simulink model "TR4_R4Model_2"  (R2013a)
settings: Solver=ode45  StartTime=0  StopTime=0.1  FixedStep=1e-4
PreLoadFcn:
  | warning('off','sm:sli:setup:compile:LocalSolverNotSupported')
InitFcn:
  |  SimParam.IC = SM2_InitCondConstrFnc(RawParam,IC);
model workspace (MAT data in the model file):
  handle : class17 (value not decoded)
  handle : class17 (value not decoded)
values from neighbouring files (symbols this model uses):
  RawParam = RobotParamGather(ParamLib)    [main_TR4.m]    (also in DeltaModelMain_v2.m; main_TimeSimulation.m; MGI.m = y)
libraries: SM2_BallJointPartsLib x8, SM2_ForeArmPartsLib x8, SM2_ArmPartsLib x4, SM2_MotorPartsLib x4, ElecDriverLib x1, SM2_FramePartsLib x1, SM2_ToolPartsLib x1

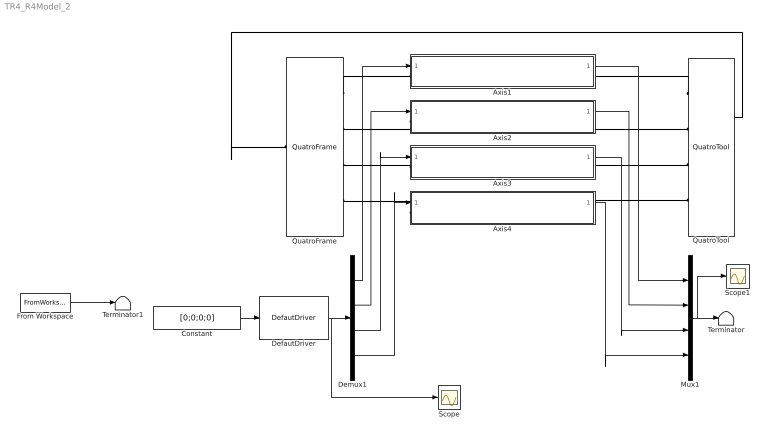
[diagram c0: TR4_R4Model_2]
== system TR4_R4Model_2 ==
  Axis1 : Subsystem
  Axis2 : Subsystem
  Axis3 : Subsystem
  Axis4 : Subsystem
  Constant : Constant  Value=[0;0;0;0]
  DefautDriver : ElecDriverLib/DefautDriver  VariantControl=driverVarDefault
  Demux1 : Demux
  From Workspace : FromWorkspace  VariableName=simin  SampleTime=0
  Mux1 : Mux
  QuatroFrame : SM2_FramePartsLib/QuatroFrame
  QuatroTool : SM2_ToolPartsLib/QuatroTool
  Scope : Scope
  Scope1 : Scope
  Terminator : Terminator
  Terminator1 : Terminator
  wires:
  Axis1/1(Alpha) -> Mux1/1
  Axis2/1(Alpha) -> Mux1/2
  Axis4/1(Alpha) -> Mux1/4
  Axis3/1(Alpha) -> Mux1/3
  Constant/1 -> DefautDriver/1
  From Workspace/1 -> Terminator1/1
  DefautDriver/1 -> Scope/1, Demux1/1
  Demux1/1 -> Axis1/1(Torque)
  Demux1/2 -> Axis2/1(Torque)
  Demux1/3 -> Axis3/1(Torque)
  Demux1/4 -> Axis4/1(Torque)
  Mux1/1 -> Scope1/1, Terminator/1
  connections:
  QuatroFrame/RConn1 -- Axis1/LConn1
  Axis2/LConn1 -- QuatroFrame/RConn2
  Axis3/LConn1 -- QuatroFrame/RConn3
  Axis3/RConn1 -- QuatroTool/RConn3
  Axis2/RConn1 -- QuatroTool/RConn2
  QuatroTool/RConn1 -- Axis1/RConn1
  QuatroTool/LConn1 -- QuatroFrame/LConn1
  Axis4/LConn1 -- QuatroFrame/RConn4
  Axis4/RConn1 -- QuatroTool/RConn4

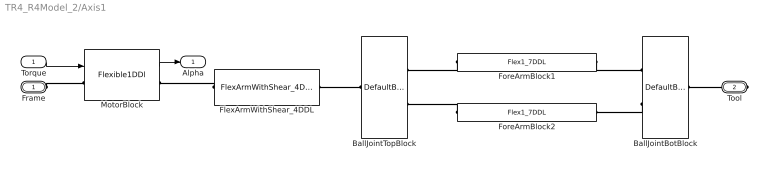
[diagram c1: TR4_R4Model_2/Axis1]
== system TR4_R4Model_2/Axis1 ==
  Torque : Inport
  BallJointBotBlock : SM2_BallJointPartsLib/DefaultBallJointBotPair
  BallJointTopBlock : SM2_BallJointPartsLib/DefaultBallJointTopPair
  FlexArmWithShear_4DDL : SM2_ArmPartsLib/FlexArmWithShear_4DDL  VariantControl=armVarFlex1_2ddl
  ForeArmBlock1 : SM2_ForeArmPartsLib/Flex1_7DDL  VariantControl=foreArmVarFlex1_7ddl
  ForeArmBlock2 : SM2_ForeArmPartsLib/Flex1_7DDL  VariantControl=foreArmVarFlex1_7ddl
  MotorBlock : SM2_MotorPartsLib/Flexible1DDl  VariantControl=motorVarFlex1
      link override Revolute Joint: ClassName=RevoluteJoint  SenseConstraintForceX=off  SenseConstraintForceY=off  SenseConstraintForceZ=off  SenseConstraintTorqueX=off  SenseConstraintTorqueY=off  SenseConstraintTorqueZ=off  ConstraintWrenchDir=FollowerOnBase  ConstraintWrenchFrame=BaseFrame  EquilibriumPosition=SimParam.Motor.Alpha(AxisID)  EquilibriumPositionUnits=rad  SpringStiffness=SimParam.Motor.kSup  SpringStiffnessUnits=N*m/rad  DampingCoefficient=SimParam.Motor.c  DampingCoefficientUnits=N*m/(rad/s)  ActuationMode=TorqueForceActuation  SensePosition=on  SenseVelocity=off  SenseAcceleration=off  SenseTorqueForce=off  PositionTargetValue=SimParam.Motor.Alpha(AxisID)  PositionTargetValueUnits=rad  PositionTargetSpecify=on  PositionTargetPriority=High  VelocityTargetValue=0  VelocityTargetValueUnits=rad/s  VelocityTargetSpecify=on  VelocityTargetPriority=High  BlockFunction=simmechanics.library.joints.revolute_joint
  Frame : PMIOPort  Port=1  Side=Left
  Tool : PMIOPort  Port=2  Side=Right
  Alpha : Outport
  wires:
  Torque/1 -> MotorBlock/1
  MotorBlock/1 -> Alpha/1
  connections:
  FlexArmWithShear_4DDL/LConn1 -- MotorBlock/RConn1
  Frame/RConn1 -- MotorBlock/LConn1
  FlexArmWithShear_4DDL/RConn1 -- BallJointTopBlock/RConn1
  Tool/RConn1 -- BallJointBotBlock/RConn1
  ForeArmBlock2/LConn1 -- BallJointTopBlock/LConn2
  ForeArmBlock1/LConn1 -- BallJointTopBlock/LConn1
  ForeArmBlock1/RConn1 -- BallJointBotBlock/LConn1
  BallJointBotBlock/LConn2 -- ForeArmBlock2/RConn1

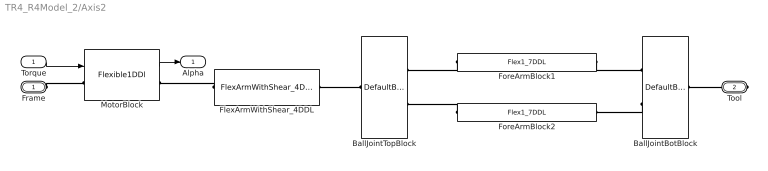
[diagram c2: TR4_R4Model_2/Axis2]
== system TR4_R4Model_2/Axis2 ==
  Torque : Inport
  BallJointBotBlock : SM2_BallJointPartsLib/DefaultBallJointBotPair
  BallJointTopBlock : SM2_BallJointPartsLib/DefaultBallJointTopPair
  FlexArmWithShear_4DDL : SM2_ArmPartsLib/FlexArmWithShear_4DDL  VariantControl=armVarFlex1_2ddl
  ForeArmBlock1 : SM2_ForeArmPartsLib/Flex1_7DDL  VariantControl=foreArmVarFlex1_7ddl
  ForeArmBlock2 : SM2_ForeArmPartsLib/Flex1_7DDL  VariantControl=foreArmVarFlex1_7ddl
  MotorBlock : SM2_MotorPartsLib/Flexible1DDl  VariantControl=motorVarFlex1
      link override Revolute Joint: ClassName=RevoluteJoint  SenseConstraintForceX=off  SenseConstraintForceY=off  SenseConstraintForceZ=off  SenseConstraintTorqueX=off  SenseConstraintTorqueY=off  SenseConstraintTorqueZ=off  ConstraintWrenchDir=FollowerOnBase  ConstraintWrenchFrame=BaseFrame  EquilibriumPosition=SimParam.Motor.Alpha(AxisID)  EquilibriumPositionUnits=rad  SpringStiffness=SimParam.Motor.kSup  SpringStiffnessUnits=N*m/rad  DampingCoefficient=SimParam.Motor.c  DampingCoefficientUnits=N*m/(rad/s)  ActuationMode=TorqueForceActuation  SensePosition=on  SenseVelocity=off  SenseAcceleration=off  SenseTorqueForce=off  PositionTargetValue=SimParam.Motor.Alpha(AxisID)  PositionTargetValueUnits=rad  PositionTargetSpecify=on  PositionTargetPriority=High  VelocityTargetValue=0  VelocityTargetValueUnits=rad/s  VelocityTargetSpecify=on  VelocityTargetPriority=High  BlockFunction=simmechanics.library.joints.revolute_joint
  Frame : PMIOPort  Port=1  Side=Left
  Tool : PMIOPort  Port=2  Side=Right
  Alpha : Outport
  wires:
  Torque/1 -> MotorBlock/1
  MotorBlock/1 -> Alpha/1
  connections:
  FlexArmWithShear_4DDL/LConn1 -- MotorBlock/RConn1
  Frame/RConn1 -- MotorBlock/LConn1
  FlexArmWithShear_4DDL/RConn1 -- BallJointTopBlock/RConn1
  Tool/RConn1 -- BallJointBotBlock/RConn1
  ForeArmBlock2/LConn1 -- BallJointTopBlock/LConn2
  ForeArmBlock1/LConn1 -- BallJointTopBlock/LConn1
  ForeArmBlock1/RConn1 -- BallJointBotBlock/LConn1
  BallJointBotBlock/LConn2 -- ForeArmBlock2/RConn1

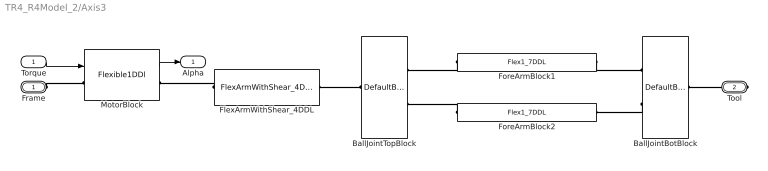
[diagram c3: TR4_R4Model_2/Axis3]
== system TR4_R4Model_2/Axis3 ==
  Torque : Inport
  BallJointBotBlock : SM2_BallJointPartsLib/DefaultBallJointBotPair
  BallJointTopBlock : SM2_BallJointPartsLib/DefaultBallJointTopPair
  FlexArmWithShear_4DDL : SM2_ArmPartsLib/FlexArmWithShear_4DDL  VariantControl=armVarFlex1_2ddl
  ForeArmBlock1 : SM2_ForeArmPartsLib/Flex1_7DDL  VariantControl=foreArmVarFlex1_7ddl
  ForeArmBlock2 : SM2_ForeArmPartsLib/Flex1_7DDL  VariantControl=foreArmVarFlex1_7ddl
  MotorBlock : SM2_MotorPartsLib/Flexible1DDl  VariantControl=motorVarFlex1
      link override Revolute Joint: ClassName=RevoluteJoint  SenseConstraintForceX=off  SenseConstraintForceY=off  SenseConstraintForceZ=off  SenseConstraintTorqueX=off  SenseConstraintTorqueY=off  SenseConstraintTorqueZ=off  ConstraintWrenchDir=FollowerOnBase  ConstraintWrenchFrame=BaseFrame  EquilibriumPosition=SimParam.Motor.Alpha(AxisID)  EquilibriumPositionUnits=rad  SpringStiffness=SimParam.Motor.kSup  SpringStiffnessUnits=N*m/rad  DampingCoefficient=SimParam.Motor.c  DampingCoefficientUnits=N*m/(rad/s)  ActuationMode=TorqueForceActuation  SensePosition=on  SenseVelocity=off  SenseAcceleration=off  SenseTorqueForce=off  PositionTargetValue=SimParam.Motor.Alpha(AxisID)  PositionTargetValueUnits=rad  PositionTargetSpecify=on  PositionTargetPriority=High  VelocityTargetValue=0  VelocityTargetValueUnits=rad/s  VelocityTargetSpecify=on  VelocityTargetPriority=High  BlockFunction=simmechanics.library.joints.revolute_joint
  Frame : PMIOPort  Port=1  Side=Left
  Tool : PMIOPort  Port=2  Side=Right
  Alpha : Outport
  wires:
  Torque/1 -> MotorBlock/1
  MotorBlock/1 -> Alpha/1
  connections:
  FlexArmWithShear_4DDL/LConn1 -- MotorBlock/RConn1
  Frame/RConn1 -- MotorBlock/LConn1
  FlexArmWithShear_4DDL/RConn1 -- BallJointTopBlock/RConn1
  Tool/RConn1 -- BallJointBotBlock/RConn1
  ForeArmBlock2/LConn1 -- BallJointTopBlock/LConn2
  ForeArmBlock1/LConn1 -- BallJointTopBlock/LConn1
  ForeArmBlock1/RConn1 -- BallJointBotBlock/LConn1
  BallJointBotBlock/LConn2 -- ForeArmBlock2/RConn1

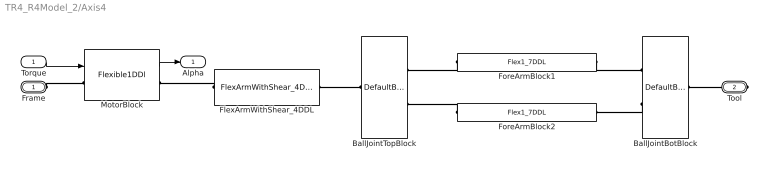
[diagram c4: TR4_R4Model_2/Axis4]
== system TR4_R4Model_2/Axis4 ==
  Torque : Inport
  BallJointBotBlock : SM2_BallJointPartsLib/DefaultBallJointBotPair
  BallJointTopBlock : SM2_BallJointPartsLib/DefaultBallJointTopPair
  FlexArmWithShear_4DDL : SM2_ArmPartsLib/FlexArmWithShear_4DDL  VariantControl=armVarFlex1_2ddl
  ForeArmBlock1 : SM2_ForeArmPartsLib/Flex1_7DDL  VariantControl=foreArmVarFlex1_7ddl
  ForeArmBlock2 : SM2_ForeArmPartsLib/Flex1_7DDL  VariantControl=foreArmVarFlex1_7ddl
  MotorBlock : SM2_MotorPartsLib/Flexible1DDl  VariantControl=motorVarFlex1
      link override Revolute Joint: ClassName=RevoluteJoint  SenseConstraintForceX=off  SenseConstraintForceY=off  SenseConstraintForceZ=off  SenseConstraintTorqueX=off  SenseConstraintTorqueY=off  SenseConstraintTorqueZ=off  ConstraintWrenchDir=FollowerOnBase  ConstraintWrenchFrame=BaseFrame  EquilibriumPosition=SimParam.Motor.Alpha(AxisID)  EquilibriumPositionUnits=rad  SpringStiffness=SimParam.Motor.kSup  SpringStiffnessUnits=N*m/rad  DampingCoefficient=SimParam.Motor.c  DampingCoefficientUnits=N*m/(rad/s)  ActuationMode=TorqueForceActuation  SensePosition=on  SenseVelocity=off  SenseAcceleration=off  SenseTorqueForce=off  PositionTargetValue=SimParam.Motor.Alpha(AxisID)  PositionTargetValueUnits=rad  PositionTargetSpecify=on  PositionTargetPriority=High  VelocityTargetValue=0  VelocityTargetValueUnits=rad/s  VelocityTargetSpecify=on  VelocityTargetPriority=High  BlockFunction=simmechanics.library.joints.revolute_joint
  Frame : PMIOPort  Port=1  Side=Left
  Tool : PMIOPort  Port=2  Side=Right
  Alpha : Outport
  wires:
  Torque/1 -> MotorBlock/1
  MotorBlock/1 -> Alpha/1
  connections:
  FlexArmWithShear_4DDL/LConn1 -- MotorBlock/RConn1
  Frame/RConn1 -- MotorBlock/LConn1
  FlexArmWithShear_4DDL/RConn1 -- BallJointTopBlock/RConn1
  Tool/RConn1 -- BallJointBotBlock/RConn1
  ForeArmBlock2/LConn1 -- BallJointTopBlock/LConn2
  ForeArmBlock1/LConn1 -- BallJointTopBlock/LConn1
  ForeArmBlock1/RConn1 -- BallJointBotBlock/LConn1
  BallJointBotBlock/LConn2 -- ForeArmBlock2/RConn1
